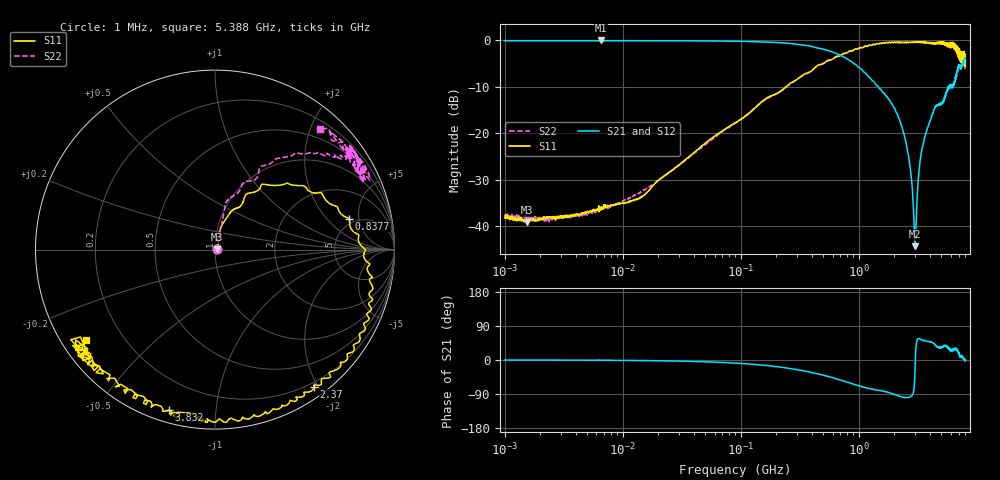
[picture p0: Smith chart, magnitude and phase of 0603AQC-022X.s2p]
!s-Parameter Generated by FASTRON Sdn. Bhd.
!FASTRON P/N : 0603AQC-022X
!Keysight Technologies: E5071C_MY46733604_B.14.02
!Date: Thu Jun 25 13:52:31 2026
!Version  :Rev00  Thu Jun 25 13:52:31 2026
!Data & Calibration Information:
!Freq  S11:SOLT2(ON)  S21:SOLT2(ON)  S12:SOLT2(ON)  S22:SOLT2(ON)
!PortZ  Port1:50+j0  Port2:50+j0
!When reading reference impedance value at option line is always used.
! Remarks : This data is being provided solely for informational purposes.
# Hz S dB R 50
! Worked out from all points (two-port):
!   1601 points, 1 MHz to 8 GHz, reference 50 ohm
!   highest |S21| = -0.06 dB at 6.532 MHz (marker M1); lowest = -44.3 dB at 3 GHz (marker M2)
!   |S21| within 3 dB of the highest: start of sweep to 674.7 MHz
!   lowest |S11| = -39.2 dB at 1.541 MHz (marker M3), VSWR 1.02, Z = 51.1 + j0.152 ohm
!   |S11| at or under -10 dB: start of sweep to 241.2 MHz
!   |S22| runs from -39.0 to -0.4 dB; largest |S21 - S12| = 0.0097
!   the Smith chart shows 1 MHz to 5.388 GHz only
!   S11 on the Smith chart (normalised r, x): 1 MHz: 1.03, +0.00; 837.7 MHz: 4.40, +3.68; 2.37 GHz: 0.14, -1.94; 3.832 GHz: 0.06, -0.75; 5.388 GHz: 0.07, -0.31
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1000000  -38.10 3.9  -0.12 -0.1  -0.11 -0.1  -37.70 6.4
1541011  -39.20 7.8  -0.11 -0.2  -0.10 -0.2  -37.80 2.2
4479405  -37.30 26.4  -0.12 -0.5  -0.12 -0.5  -37.60 28.6
6531720  -36.20 33.0  -0.06 -0.6  -0.08 -0.5  -36.50 37.9
1.388866e7  -33.90 52.7  -0.12 -1.4  -0.12 -1.4  -32.90 54.6
2.00676e7  -30.10 58.4  -0.13 -1.9  -0.13 -1.9  -30.10 66.8
8.994653e7  -17.80 75.2  -0.22 -8.2  -0.23 -8.2  -17.80 74.6
4.006501e8  -6.58 50.1  -1.34 -33.4  -1.34 -33.4  -6.45 59.9
8.377436e8  -2.31 13.0  -4.38 -60.1  -4.38 -60.2  -2.45 45.6
1.272209e9  -1.14 -10.9  -8.38 -76.6  -8.39 -76.8  -1.06 34.8
1.7949e9  -0.48 -31.3  -12.70 -85.5  -12.80 -85.7  -0.50 36.4
2.369519e9  -0.51 -54.3  -19.50 -98.3  -19.60 -98.3  -0.47 30.9
2.692309e9  -0.40 -65.3  -26.30 -97.6  -26.40 -97.6  -0.46 35.8
2.927065e9  -0.45 -72.7  -38.00 -79.3  -37.90 -79.6  -0.47 37.0
3.000426e9  -0.36 -75.8  -44.30 -16.9  -44.50 -15.8  -0.46 37.7
3.345355e9  -0.44 -89.1  -25.10 54.6  -25.10 54.8  -0.46 30.5
3.831807e9  -0.62 -106.0  -18.80 49.3  -18.80 49.2  -0.60 31.5
4.744521e9  -0.39 -138.0  -14.00 32.9  -14.00 32.6  -0.69 24.9
5.388334e9  -1.11 -145.0  -11.80 39.0  -11.80 38.7  -1.00 48.8
6.419251e9  -0.60 -172.0  -9.64 26.2  -9.61 25.8  -1.30 49.1
7.190348e9  -2.56 150.0  -5.80 7.2  -5.80 6.4  -3.30 40.2
8e9  -2.99 145.0  -4.29 -2.4  -4.32 -3.0  -4.27 53.7
